(* Logix 5000 AddOnInstructionDefinition export MAB_Yaskawa; software revision 17.00 *)

TYPE Yaskawa_EIP_Servo :   // Yaskawa SigmaLogic Axis Structure v2.4.0
STRUCT
   O : Yaskawa_OUT_to_Servo;
   I : Yaskawa_IN_from_Servo;
   AOI_SB : Yaskawa_AOI_Status_Bits;
END_STRUCT
END_TYPE

TYPE Yaskawa_OUT_to_Servo :   // Structure of data sent out to the Yaskawa SigmaLogic controller v2.4.0
STRUCT
   b00_ServoOn : BOOL;   // Servo On
   b01_Stop : BOOL;   // Stops All Current Motion in Progress
   b02_Home : BOOL;   // Start Homing Process
   b03_MoveStart1 : BOOL;   // Start Current Motion
   b06_SuperImpose : BOOL;
   b07_ServoAlarmReset : BOOL;   // Servo Alarm Reset
   b08_ControllerAlarmReset : BOOL;   // SigmaLogic Alarm Reset
   b09_MoveStart2 : BOOL;   // Start Second Motion (Blended Move)
   b10_MoveAbort : BOOL;   // Abort Current Move
   b11_MovePause : BOOL;   // Pause Current Move
   b12_SeqPause : BOOL;   // Indexing Sequence Pause
   b13_SeqResume : BOOL;   // Indexing Sequence Resume
   b14_SeqCancel : BOOL;   // Indexing Sequence Cancel
   b15_AbsEncoderReset : BOOL;   // Absolute Encoder Reset
   b16_SeqStart : BOOL;   // Start Indexing Sequence
   b17_SeqEditSpeed : BOOL;   // Enter Edit Speed
   b18_SeqEditDistance : BOOL;   // Enter Distance Edit
   b19_PLSEnable : BOOL;   // Enable PLS execution
   b20_PLSActivateOutput1 : BOOL;   // Activate PLS output1 switch logic
   b21_PLSActivateOutput2 : BOOL;   // Activate PLS output2 switch logic
   b22_PLSActivateOutput3 : BOOL;   // Activate PLS output3 switch logic
   b23_PLSActivateOutput4 : BOOL;   // Activate PLS output4 switch logic
   b24_SetClock : BOOL;   // Set the remote controller clock with data provided by the PLC
   RebootController : BOOL;
   UseExternalEncoder : BOOL;   // Use External Encoder when executing MAHSP_Yaskawa
   b32_HeatbeatAnswer : BOOL;   // Heartbeat Answer
   BrakeBypassRequest : BOOL;
   SetFwdTorqueLimit : BOOL;
   SetRevTorqueLimit : BOOL;
   TorqueLimit : DINT;
   TorqueRamp : DINT;
   HomeMethod : INT;
   HomeSpeed : DINT;
   HomeAccDec : DINT;   // Home Move Acceleration/Deceleration Rate
   HomeBackOffDistance : DINT;
   HomeCreepSpeed : DINT;
   HomeCreepDistanceLimit : DINT;
   HomeCreepTimeLimit : DINT;
   HomeOffsetDistance : DINT;
   HomeOffsetSpeed : DINT;
   HomePostion : DINT;
   HomeTorque : DINT;
   HomeInputNo : DINT;
   HomeApproachTimeLimit : DINT;
   HomeApproachDistLimit : DINT;
   HomeDirection : INT;
   HomeSwitchMode : INT;
   MoveType : INT;
   MoveDirection : INT;
   MoveAccel1 : DINT;
   MoveAccel2 : DINT;
   MoveDecel1 : DINT;
   MoveDecel2 : DINT;
   MoveSpeed1 : DINT;
   MoveSpeed2 : DINT;
   MoveDistance1 : DINT;
   MoveDistance2 : DINT;
   MovePosition1 : DINT;
   MovePosition2 : DINT;
   RegistrationDistance : DINT;
   GearNumerator : DINT;
   GearDenominator : DINT;
   SuperImposeDistance : DINT;
   Resolution : INT;
   RegistrationDirection : INT;
   TuningLevel : INT;
   SequenceStep : INT;   // Staring Sequence Step Number
   SequenceEditStep : INT;   // Sequence Step Number to Edit
   FlagCommandBits1 : DINT;   // Flag Commands. 1..64 are General Flags, Bits 0..31 correspond to Flag 1..32
   FlagCommandBits2 : DINT;   // Flag Commands cont. 1..64 are General Flags, Bits 0..31 correspond to Flag 33..64
   DigitalOutCommandBits : DINT;   // Digital Output commands. Bits 0-7 correspond to CN13 Digital Outputs 0-7, used as Flag 73-80. Bits 8-10 correspond to CN1 Digital Outputs 0-2 used as Flag 88-90"
   SequenceEditSpeed : DINT;
   SequenceEditDistance : DINT;
   FeedRateOverride : INT;
   HSI_Enable : BOOL;
   HSI_MoveMode : BOOL;   // 0=Relative; 1=Moves per Cycle
   HSI_CalcMethod : BOOL;   // 0=Accel/Decel; 1=Time
   HSI_MoveDirection : BOOL;   // 0 = Negative; 1 = Positive
   HSI_TriggerFlag : INT;
   HSI_MovingFlag : INT;
   HSI_DwellingFlag : INT;
   HSI_DoneFlag : INT;
   HSI_MoveType : INT;   // 0=Single; 1=Repeat; 2=Repeat "x" times
   HSI_RepeatNumber : INT;
   HSI_Distance : DINT;
   HSI_Speed : DINT;
   HSI_Accel : DINT;
   HSI_MoveTime : DINT;
   HSI_DwellTime : DINT;
   PLS_OutputFlag1 : INT;
   PLS_OutputFlag2 : INT;
   PLS_OutputFlag3 : INT;
   PLS_OutputFlag4 : INT;
   PLS_OnPosition1 : DINT;
   PLS_OffPosition1 : DINT;
   PLS_OnPosition2 : DINT;
   PLS_OffPosition2 : DINT;
   PLS_OnPosition3 : DINT;
   PLS_OffPosition3 : DINT;
   PLS_OnPosition4 : DINT;
   PLS_OffPosition4 : DINT;
   PLS_OnCompensation1 : INT;
   PLS_OffCompensation1 : INT;
   PLS_OnCompensation2 : INT;
   PLS_OffCompensation2 : INT;
   PLS_OnCompensation3 : INT;
   PLS_OffCompensation3 : INT;
   PLS_OnCompensation4 : INT;
   PLS_OffCompensation4 : INT;
   RTC_Year : INT;
   RTC_Month : INT;
   RTC_Day : INT;
   RTC_Hour : INT;
   RTC_Min : INT;
   RTC_Sec : INT;
   StopDecel : DINT;
   AnalogOutput : INT;   // CN13, AO_01 [mV]
END_STRUCT
END_TYPE

TYPE Yaskawa_AOI_Status_Bits :   // Internal bits used to interlock Yaskawa AOI execution. v2.4.0
STRUCT
   MAM : BOOL;   // Move AOI Active
   MAJ : BOOL;   // Jog AOI Active
   MAB : BOOL;   // Blending AOI Active
   MAG : BOOL;   // Gearing AOI Active
   MAHSP : BOOL;   // Home SetPoint AOI Active
   MAH : BOOL;   // Homing AOI Active
   MSQE : BOOL;   // Sequence Edit AOI Active
   MSQR : BOOL;   // Sequence Run AOI Active
   MHSI : BOOL;   // High Speed Index AOI Active
   MSO : BOOL;   // Servo On
   MSF : BOOL;   // Servo Off
   MAFR : BOOL;   // Fault Reset
   MAS : BOOL;   // Servo Abort
   MTRQ : BOOL;   // Torque Mode Active
   MPLS : BOOL;   // PLS Active
   MCLK : BOOL;   // SetClock Active
   MSTL : BOOL;   // Set Torque Limit Active
   AOI_Permissive : BOOL;   // Permissive to Execute an AOI
END_STRUCT
END_TYPE

TYPE Yaskawa_IN_from_Servo :   // Structure of data coming from the Yaskawa SigmaLogic controller. v2.4.0
STRUCT
   AlarmText : STRING;   // ServoPack Alarm Code plus Text Description
   b00_Heartbeat : BOOL;
   b01_Alarm : BOOL;   // ServoPack Alarm
   b02_Warning : BOOL;   // ServoPack Warning
   b03_Ready : BOOL;   // ServoPack Ready
   b04_Enabled : BOOL;   // ServoPack Enabled ("Servo On")
   b05_StopComplete : BOOL;
   b06_HomeComplete : BOOL;
   b07_HomeBusy : BOOL;
   b08_HomeActive : BOOL;
   b09_HomeAborted : BOOL;
   b10_HomeError : BOOL;
   b11_MoveAbsComplete : BOOL;
   b12_MoveAbsBusy : BOOL;
   b13_MoveAbsActive : BOOL;
   b14_MoveAbsAborted : BOOL;
   b15_MoveAbsError : BOOL;
   b16_MoveRelComplete : BOOL;
   b17_MoveRelBusy : BOOL;
   b18_MoveRelActive : BOOL;
   b19_MoveRelAborted : BOOL;
   b20_MoveRelError : BOOL;
   b21_JogAtSpeed : BOOL;
   b22_JogBusy : BOOL;
   b23_JogActive : BOOL;
   b24_JogAborted : BOOL;
   b25_JogError : BOOL;
   b26_GearInSync : BOOL;
   b27_GearBusy : BOOL;
   b28_GearActive : BOOL;
   b29_GearAborted : BOOL;
   b30_GearError : BOOL;
   b32_MoveSuperComplete : BOOL;
   b33_MoveSuperBusy : BOOL;
   b34_MoveSuperActive : BOOL;
   b35_MoveSuperAborted : BOOL;
   b36_MoveSuperError : BOOL;
   b37_PowerCycleRequired : BOOL;
   b38_MoveBlend1Complete : BOOL;
   b39_MoveBlend1Busy : BOOL;
   b40_MoveBlend1Active : BOOL;
   b41_MoveBlend1Abort : BOOL;
   b42_MoveBlend1Error : BOOL;
   b43_MoveBlend2Complete : BOOL;
   b44_MoveBlend2Busy : BOOL;
   b45_MoveBlend2Active : BOOL;
   b46_MoveBlend2Abort : BOOL;
   b47_MoveBlend2Error : BOOL;
   b48_RegComplete : BOOL;
   b49_RegBusy : BOOL;
   b50_RegActive : BOOL;
   b51_RegAborted : BOOL;
   b52_RegError : BOOL;
   b53_ResetAbsEncoderActive : BOOL;
   b54_ResetAbsEncoderBusy : BOOL;
   b55_ResetAbsEncoderDone : BOOL;
   b56_ResetAbsEncoderError : BOOL;
   b57_SeqRunning : BOOL;
   b58_RegSensorNotReached : BOOL;
   b59_SeqEditError : BOOL;
   b60_SeqEditDone : BOOL;
   b61_TorqueAtTorque : BOOL;
   b62_TorqueBusy : BOOL;
   b63_TorqueActive : BOOL;
   b64_TorqueAborted : BOOL;
   b65_TorqueError : BOOL;
   b66_ControllerAlarm : BOOL;
   b67_ApplicationError : BOOL;
   b68_AxisAtStandStill : BOOL;
   b69_TestModeActive : BOOL;
   b70_ServoParamsOK : BOOL;
   b71_SetFwdTorqueLimitDone : BOOL;
   b72_SetRevTorqueLimitDone : BOOL;
   Position : DINT;
   Speed : DINT;
   Torque : DINT;
   HomeErrorID : INT;
   MoveAbsErrorID : INT;
   MoveRelErrorID : INT;
   JogErrorID : INT;
   GearErrorID : INT;
   MoveSuperErrorID : INT;
   ServoAlarmID : INT;
   ServoWarningID : INT;
   ControllerAlarmID : DINT;
   AxisGenAlarmID : DINT;
   MoveBlend1ErrorID : INT;
   MoveBlend2ErrorID : INT;
   ResetAbsEncoderErrorID : INT;
   FunctionBlockErrorID : INT;
   TorqueErrorID : INT;
   RegErrorID : INT;
   SeqCurrentStep : INT;
   FlagStatusBit1 : DINT;   // Flag Status. 1..64 are General Flags, Bits 0..31 correspond to Flag 1..32
   FlagStatusBit2 : DINT;   // Flag Status cont. 1..64 are General Flags, Bits 0..31 correspond to Flag 33..64
   IOStatusBits : DINT;   // Digital IO Status. Bits 0-7, CN13 Inputs 0-7, Used as Flag 65-72. Bits 8-15, CN13 Outputs 0-7, Used as Flag 73-80. Bits 16-22, CN1 Inputs 0-6, Used as Flag 81-87. Bits 23-25, CN1 Outputs 0-4, Used as Flag 88-92.
   HSI_Moving : BOOL;
   HSI_Dwelling : BOOL;
   HSI_Done : BOOL;
   HSI_Busy : BOOL;
   HSI_Error : BOOL;
   HSI_ErrorCode : INT;
   PLS_Running : BOOL;
   PLS_SwitchStatus1 : BOOL;
   PLS_SwitchStatus2 : BOOL;
   PLS_SwitchStatus3 : BOOL;
   PLS_SwitchStatus4 : BOOL;
   PLS_Busy : BOOL;
   PLS_Error : BOOL;
   PLS_ErrorCode : INT;
   SetClock_Done : BOOL;
   SetClock_Busy : BOOL;
   SetClock_Error : BOOL;
   SetClock_ErrorID : INT;
   SoftwareVersion : DINT;
   FirmwareVersion : DINT;
   CommandedPos : DINT;
   CommandedPosNonCyc : DINT;
   CommandedSpeed : DINT;
   Clock_Year : INT;
   Clock_Month : INT;
   Clock_Day : INT;
   Clock_Hour : INT;
   Clock_Minute : INT;
   Clock_Second : INT;
   AnalogInput : REAL;   // CN13, AI_01 [v]
   BrakeBypassActive : BOOL;
   ForwardTorqueLimit : DINT;
   ReverseTorqueLimit : DINT;
END_STRUCT
END_TYPE

ADD_ON_INSTRUCTION MAB_Yaskawa   (* revision 2.4 0, vendor Yaskawa America, Inc., ExecuteEnableInFalse *)
// Motion Axis Blend
// Revision note:
// 2.4.0: No function changes
// 2.3.1: Moved unlatch of AOI_ON_LOCAL to bottom of EnableInFalse routine so that outputs will be on for at least 1 scan if one-shot on EN is used.
// 2.3.0: No functional change
// 2.0.0: Improved output operation and error code reporting. Improved interlocking with embedded code.
// 1.2.0: No functional change.
// Initial Release 9/10/2014
// Help:
// This AOI provides for a 2-speed move to an absolute position. Each portion of the move has parameters for Accel, Decel, Speed and Absolute Position Target. Blend1_Position is the absolute point at which the speed will begin changing to Blend2_Speed using Blend2_Accel and Blend2_Decel.
// CAUTION:  Because the position settings represent an absolute location, a reversal in motion could occur. Use caution when entering these values.
VAR_IN_OUT
   Axis : Yaskawa_EIP_Servo; {required}
END_VAR
VAR_INPUT
   Blend1_Accel : REAL; {required}   // Acceleration for the 1st section [unit/s/s]
   Blend1_Decel : REAL; {required}   // Deceleration for the 1st section [unit/s/s]
   Blend1_Speed : REAL; {required}   // Commanded Speed for the 1st section [unit/s]
   Blend1_Position : REAL; {required}   // Absolute position for the section change point (+/- [unit])
   Blend2_Accel : REAL; {required}   // Acceleration for the 2nd section [unit/s/s]
   Blend2_Decel : REAL; {required}   // Deceleration for the 2nd section [unit/s/s]
   Blend2_Speed : REAL; {required}   // Commanded Speed for the 2nd section [unit/s]
   Blend2_Position : REAL; {required}   // Final absolute position (+/- [unit])
END_VAR
VAR_OUTPUT
   EN : BOOL; {visible}   // The AOI Is Active
   B1_IP : BOOL; {visible}   // Indication that 1st section is in process
   B1_DN : BOOL; {visible}   // Indication that 1st section is completed
   B2_IP : BOOL; {visible}   // Indication that 2nd section is in process
   B2_DN : BOOL; {visible}   // Indication that 2nd section is completed
   ER : BOOL; {visible}   // There has been an Error in motion reported from the SigmaLogic servo axis
   PC : BOOL; {visible}   // The Axis has reached the end position (Process Complete)
   FLT_RDY : BOOL; {visible}   // The Servo is Not Ready
   FLT_BSY : BOOL; {visible}   // There is another AOI Active for this Axis
   MoveBlend1ErrorCode : INT; {visible}   // 1st section Move Error Code
   MoveBlend2ErrorCode : INT; {visible}   // 2nd section Move Error Code
END_VAR
VAR
   AOI_ON_LOCAL : BOOL;
   ScaleFactor : DINT;
   Finished : BOOL;   // Function is Finished
   Execute_OS : BOOL;
END_VAR

ROUTINE EnableInFalse   (* ladder *)
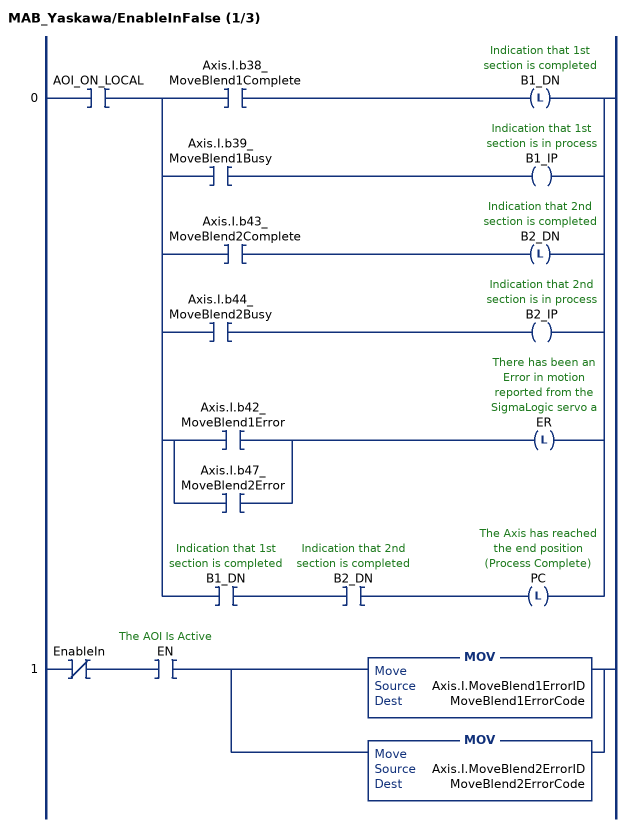
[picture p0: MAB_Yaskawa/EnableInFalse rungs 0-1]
   0: XIC(AOI_ON_LOCAL)[XIC(Axis.I.b38_MoveBlend1Complete) OTL(B1_DN) ,XIC(Axis.I.b39_MoveBlend1Busy) OTE(B1_IP) ,XIC(Axis.I.b43_MoveBlend2Complete) OTL(B2_DN) ,XIC(Axis.I.b44_MoveBlend2Busy) OTE(B2_IP) ,[XIC(Axis.I.b42_MoveBlend1Error) ,XIC(Axis.I.b47_MoveBlend2Error) ] OTL(ER) ,XIC(B1_DN) XIC(B2_DN) OTL(PC) ];
   1: XIO(EnableIn)XIC(EN)[MOV(Axis.I.MoveBlend1ErrorID,MoveBlend1ErrorCode) ,MOV(Axis.I.MoveBlend2ErrorID,MoveBlend2ErrorCode) ];
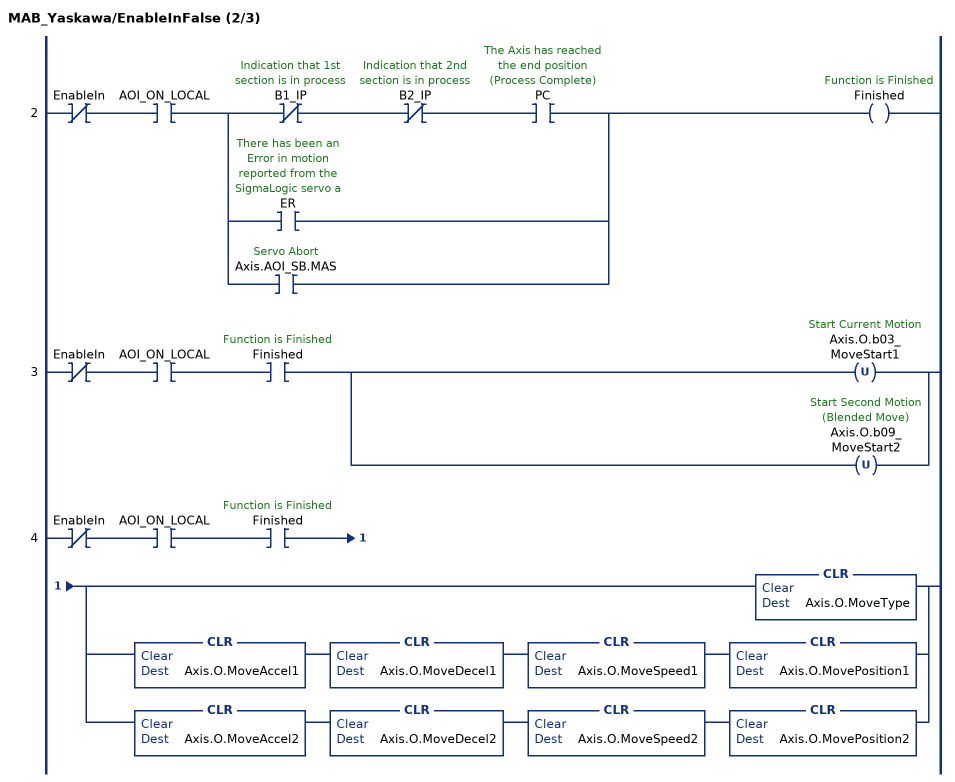
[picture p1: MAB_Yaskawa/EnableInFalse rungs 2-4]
   2: XIO(EnableIn)XIC(AOI_ON_LOCAL)[XIO(B1_IP) XIO(B2_IP) XIC(PC) ,XIC(ER) ,XIC(Axis.AOI_SB.MAS) ]OTE(Finished);
   3: XIO(EnableIn)XIC(AOI_ON_LOCAL)XIC(Finished)[OTU(Axis.O.b03_MoveStart1) ,OTU(Axis.O.b09_MoveStart2) ];
   4: XIO(EnableIn)XIC(AOI_ON_LOCAL)XIC(Finished)[CLR(Axis.O.MoveType) ,CLR(Axis.O.MoveAccel1) CLR(Axis.O.MoveDecel1) CLR(Axis.O.MoveSpeed1) CLR(Axis.O.MovePosition1) ,CLR(Axis.O.MoveAccel2) CLR(Axis.O.MoveDecel2) CLR(Axis.O.MoveSpeed2) CLR(Axis.O.MovePosition2) ];
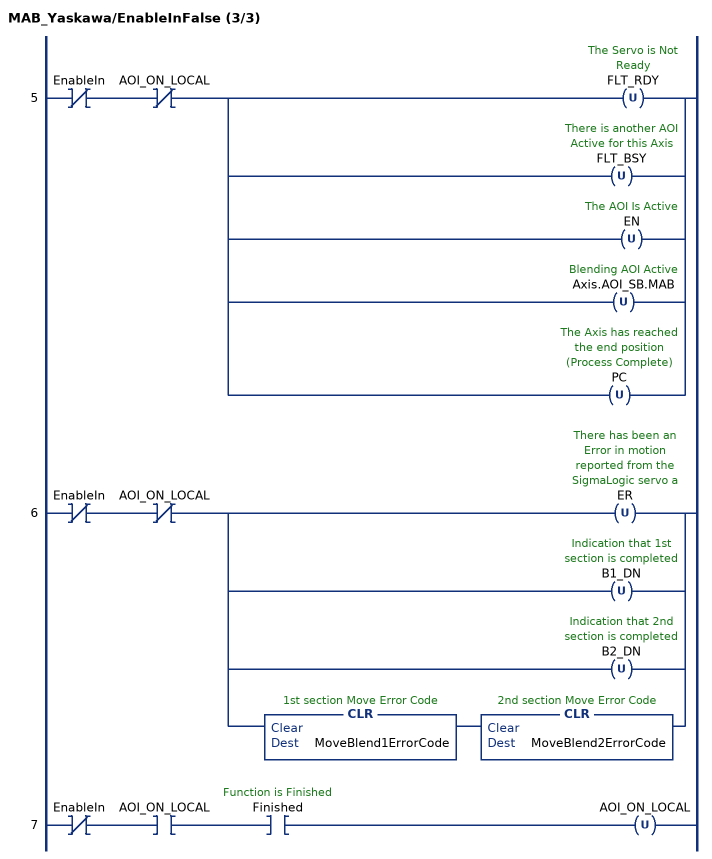
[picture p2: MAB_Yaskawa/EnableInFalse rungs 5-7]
   5: XIO(EnableIn)XIO(AOI_ON_LOCAL)[OTU(FLT_RDY) ,OTU(FLT_BSY) ,OTU(EN) ,OTU(Axis.AOI_SB.MAB) ,OTU(PC) ];
   6: XIO(EnableIn)XIO(AOI_ON_LOCAL)[OTU(ER) ,OTU(B1_DN) ,OTU(B2_DN) ,CLR(MoveBlend1ErrorCode) CLR(MoveBlend2ErrorCode) ];
   7: XIO(EnableIn)XIC(AOI_ON_LOCAL)XIC(Finished)OTU(AOI_ON_LOCAL);
END_ROUTINE

ROUTINE Logic   (* ladder *)
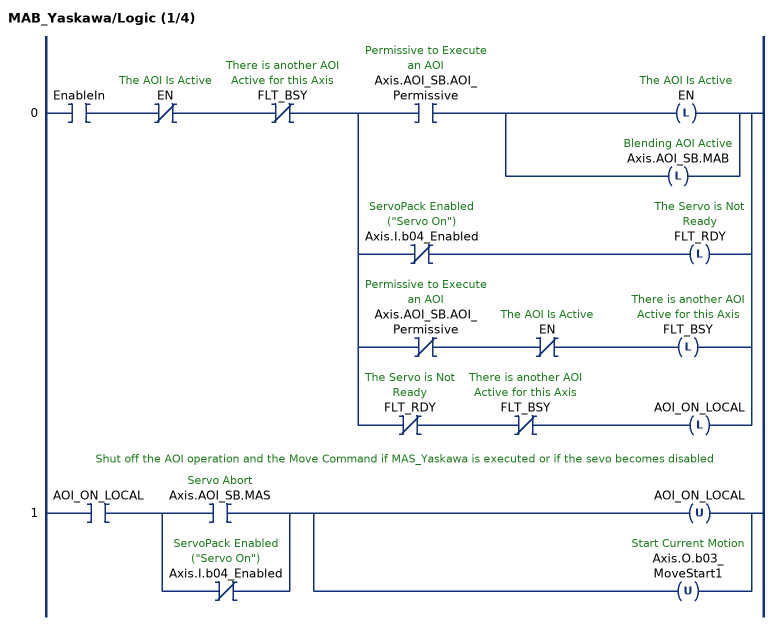
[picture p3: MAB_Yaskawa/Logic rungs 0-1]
   0: XIC(EnableIn)XIO(EN)XIO(FLT_BSY)[XIC(Axis.AOI_SB.AOI_Permissive) [OTL(EN) ,OTL(Axis.AOI_SB.MAB) ] ,XIO(Axis.I.b04_Enabled) OTL(FLT_RDY) ,XIO(Axis.AOI_SB.AOI_Permissive) XIO(EN) OTL(FLT_BSY) ,XIO(FLT_RDY) XIO(FLT_BSY) OTL(AOI_ON_LOCAL) ];
   // Shut off the AOI operation and the Move Command if MAS_Yaskawa is executed or if the sevo becomes disabled
   1: XIC(AOI_ON_LOCAL)[XIC(Axis.AOI_SB.MAS) ,XIO(Axis.I.b04_Enabled) ][OTU(AOI_ON_LOCAL) ,OTU(Axis.O.b03_MoveStart1) ];
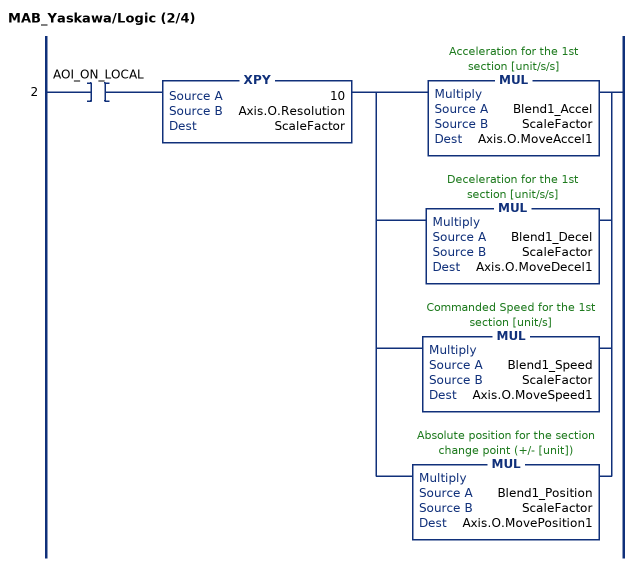
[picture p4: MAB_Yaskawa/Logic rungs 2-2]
   2: XIC(AOI_ON_LOCAL)XPY(10,Axis.O.Resolution,ScaleFactor)[MUL(Blend1_Accel,ScaleFactor,Axis.O.MoveAccel1) ,MUL(Blend1_Decel,ScaleFactor,Axis.O.MoveDecel1) ,MUL(Blend1_Speed,ScaleFactor,Axis.O.MoveSpeed1) ,MUL(Blend1_Position,ScaleFactor,Axis.O.MovePosition1) ];
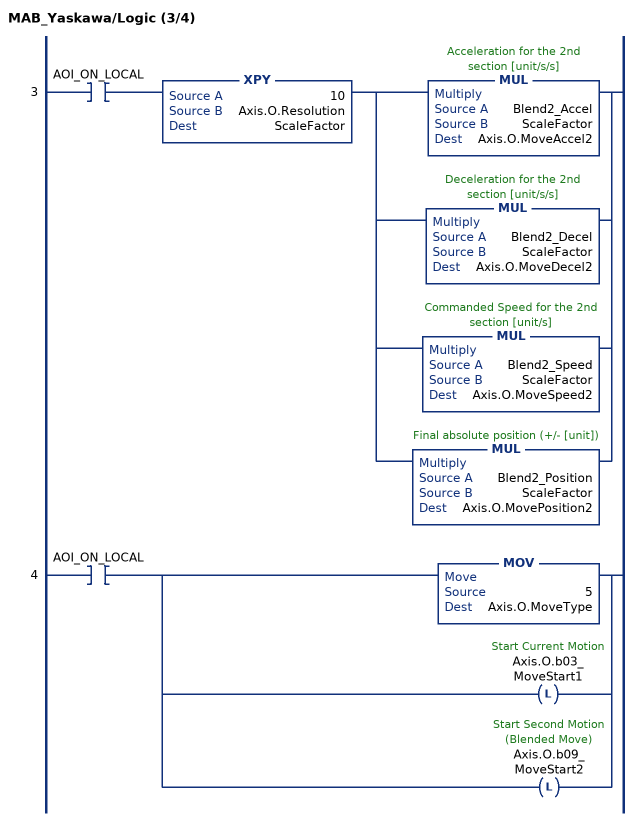
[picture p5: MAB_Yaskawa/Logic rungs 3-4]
   3: XIC(AOI_ON_LOCAL)XPY(10,Axis.O.Resolution,ScaleFactor)[MUL(Blend2_Accel,ScaleFactor,Axis.O.MoveAccel2) ,MUL(Blend2_Decel,ScaleFactor,Axis.O.MoveDecel2) ,MUL(Blend2_Speed,ScaleFactor,Axis.O.MoveSpeed2) ,MUL(Blend2_Position,ScaleFactor,Axis.O.MovePosition2) ];
   4: XIC(AOI_ON_LOCAL)[MOV(5,Axis.O.MoveType) ,OTL(Axis.O.b03_MoveStart1) ,OTL(Axis.O.b09_MoveStart2) ];
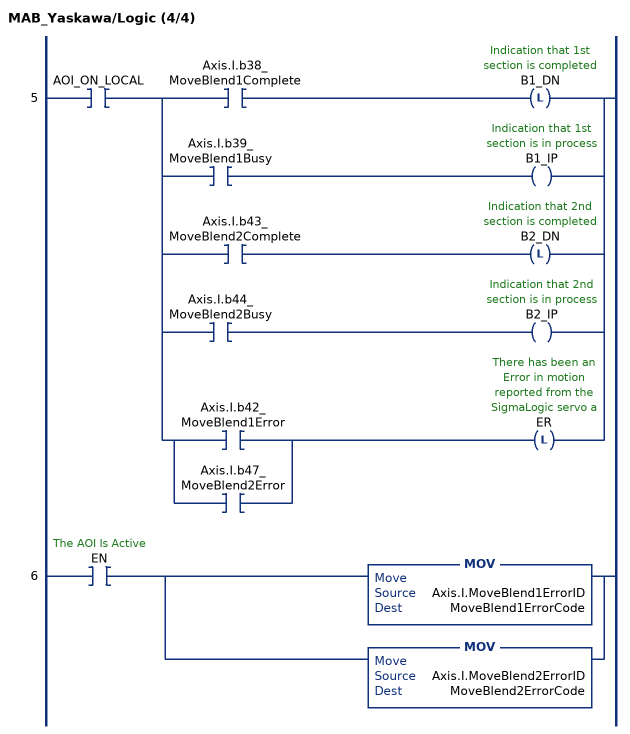
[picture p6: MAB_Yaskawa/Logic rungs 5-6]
   5: XIC(AOI_ON_LOCAL)[XIC(Axis.I.b38_MoveBlend1Complete) OTL(B1_DN) ,XIC(Axis.I.b39_MoveBlend1Busy) OTE(B1_IP) ,XIC(Axis.I.b43_MoveBlend2Complete) OTL(B2_DN) ,XIC(Axis.I.b44_MoveBlend2Busy) OTE(B2_IP) ,[XIC(Axis.I.b42_MoveBlend1Error) ,XIC(Axis.I.b47_MoveBlend2Error) ] OTL(ER) ];
   6: XIC(EN)[MOV(Axis.I.MoveBlend1ErrorID,MoveBlend1ErrorCode) ,MOV(Axis.I.MoveBlend2ErrorID,MoveBlend2ErrorCode) ];
END_ROUTINE
END_ADD_ON_INSTRUCTION
